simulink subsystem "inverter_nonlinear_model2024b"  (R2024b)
settings: Solver=VariableStepAuto  StartTime=0.0  StopTime=10.0  RelTol=1e-3
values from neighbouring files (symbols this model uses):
  Cdc = diag(Cdc1.*ones(nv,1))    [nine_bus_parameters.m]
  Cf = diag(Cf1.*ones(nv,1))    [nine_bus_parameters.m]
  F = diag(F1.*ones(nv,1))    [nine_bus_parameters.m]
  Kic = diag(Kic1.*ones(nv,1))    [nine_bus_parameters.m]
  Kiv = diag(Kiv1.*ones(nv,1))    [nine_bus_parameters.m]
  Kpc = diag(Kpc1.*ones(nv,1))    [nine_bus_parameters.m]
  Kpv = diag(Kpv1.*ones(nv,1))    [nine_bus_parameters.m]
  Lc = diag(Lc1.*ones(nv,1))    [nine_bus_parameters.m]
  Ldc = diag(Ldc1.*ones(nv,1))    [nine_bus_parameters.m]
  Lf = diag(Lf1.*ones(nv,1))    [nine_bus_parameters.m]
  mp = diag(mp1.*ones(nv,1))    [nine_bus_parameters.m]
  nq = diag(nq1.*ones(nv,1))    [nine_bus_parameters.m]
  rc = diag(rc1.*ones(nv,1))    [nine_bus_parameters.m]
  rdc = diag(rdc1.*ones(nv,1))    [nine_bus_parameters.m]
  rf = diag(rf1.*ones(nv,1))    [nine_bus_parameters.m]
  Vdc = ones(num_inv,1).*Vdc(1)    [nine_bus_initial_conditions.m]    (also in nine_bus_parameters.m = Vdc1.*ones(nv,1))
  Vn = 380    [simulink_parameters_one_bus.m]    (also in nine_bus_parameters.m = 310.*ones(num_inv,1))
  Vtri = Vdc1./3    [simulink_parameters_one_bus.m]    (also in nine_bus_parameters.m = Vdc./2)
  wc = diag(wc1.*ones(nv,1))    [nine_bus_parameters.m]
  wn = ones(num_inv,1).*w01    [nine_bus_parameters.m]    (also in computeModeFrequencyDampingTable.m = abs(lambda))
  x0 = x01    [mlinearize_noninv.m]    (also in onebus_nonlinsub.m; DemoMTI_Boolean_Index_MTI.m = [0.5 0.0000]; DemoMTI_EKF.m = [1;-1;0.5]; DemoMTI_hybridSystemsTankExamples.m = 30)
libraries: slpidlib x4

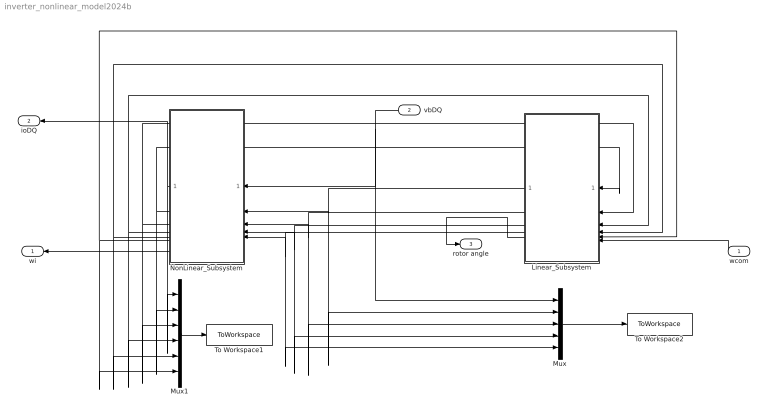
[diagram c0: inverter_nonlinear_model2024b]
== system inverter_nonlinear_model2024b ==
  wcom : Inport
  vbDQ : Inport  Port=2  OutDataTypeStr=double  PortDimensions=2
  Linear_Subsystem : Subsystem
  Mux : Mux  Inputs=5
  Mux1 : Mux  Inputs=6
  NonLinear_Subsystem : Subsystem
  To Workspace1 : ToWorkspace  VariableName=output_data  SaveFormat=Timeseries  SampleTime=-1
  To Workspace2 : ToWorkspace  VariableName=input_data  SaveFormat=Timeseries  SampleTime=-1
  wi : Outport
  ioDQ : Outport  Port=2
  rotor angle : Outport  Port=3
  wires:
  wcom/1 -> Linear_Subsystem/6(wcom)
  Linear_Subsystem/3(wi) -> Mux/4, NonLinear_Subsystem/4(wi_in)
  vbDQ/1 -> Mux/1, NonLinear_Subsystem/1(vbDQ)
  Linear_Subsystem/1(P) -> Mux/2, NonLinear_Subsystem/2(P)
  Linear_Subsystem/2(vref) -> Mux/3, NonLinear_Subsystem/3(vref)
  Linear_Subsystem/4(delta) -> Mux/5, NonLinear_Subsystem/5(delta)
  NonLinear_Subsystem/1(ioDQ) -> ioDQ/1, Mux1/1
  NonLinear_Subsystem/2(il) -> Linear_Subsystem/1(il), Mux1/2
  NonLinear_Subsystem/3(io) -> Linear_Subsystem/2(io), Mux1/3
  NonLinear_Subsystem/4(vo) -> Linear_Subsystem/3(vo), Mux1/4
  NonLinear_Subsystem/5(p) -> Mux1/5, Linear_Subsystem/4(p)
  NonLinear_Subsystem/6(q) -> Linear_Subsystem/5(q), Mux1/6
  Mux/1 -> To Workspace2/1
  NonLinear_Subsystem/7(wi_out) -> wi/1
  Linear_Subsystem/5(rotor angle) -> rotor angle/1
  Mux1/1 -> To Workspace1/1

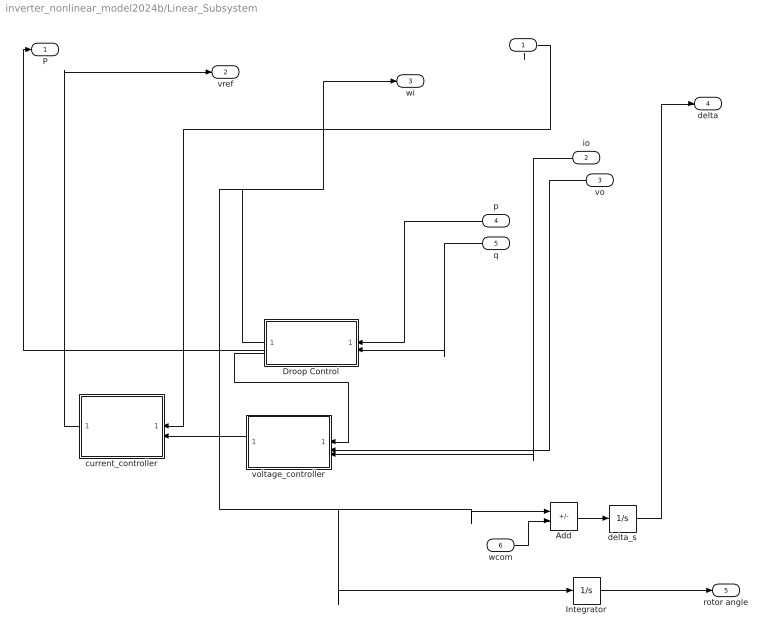
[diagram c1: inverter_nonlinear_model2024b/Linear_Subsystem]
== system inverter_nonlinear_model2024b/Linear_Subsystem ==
  il : Inport
  io : Inport  Port=2
  vo : Inport  Port=3
  p : Inport  Port=4
  q : Inport  Port=5
  wcom : Inport  Port=6
  Add : Sum  Inputs=+-
  Droop Control : Subsystem
  Integrator : Integrator  InitialCondition=2*pi*60  ZeroCross=off
  current_controller : Subsystem
  delta_s : Integrator  InitialCondition=x0(3)
  voltage_controller : Subsystem
  P : Outport
  vref : Outport  Port=2
  wi : Outport  Port=3
  delta : Outport  Port=4
  rotor angle : Outport  Port=5  VectorParamsAs1DForOutWhenUnconnected=off
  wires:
  Droop Control/1(wi) -> wi/1, Add/1, Integrator/1
  Integrator/1 -> rotor angle/1
  Droop Control/2(P) -> P/1
  Droop Control/3(voref) -> voltage_controller/1(voref)
  Add/1 -> delta_s/1
  vo/1 -> voltage_controller/2(vo)
  voltage_controller/1(iref) -> current_controller/2(ilref)
  wcom/1 -> Add/2
  p/1 -> Droop Control/1(p)
  q/1 -> Droop Control/2(q)
  il/1 -> current_controller/1(il)
  current_controller/1(vref) -> vref/1
  delta_s/1 -> delta/1
  io/1 -> voltage_controller/3(io)

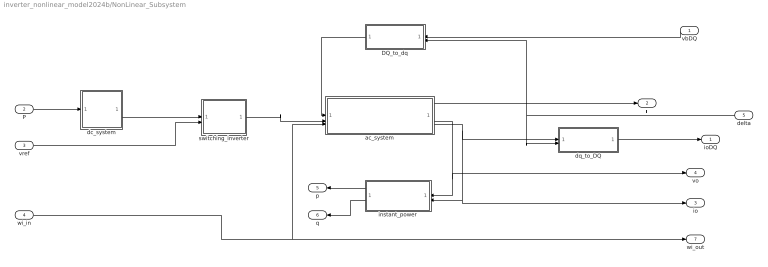
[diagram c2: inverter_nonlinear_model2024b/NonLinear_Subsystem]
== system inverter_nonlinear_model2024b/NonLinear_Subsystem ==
  vbDQ : Inport
  P : Inport  Port=2
  vref : Inport  Port=3
  wi_in : Inport  Port=4
  delta : Inport  Port=5
  DQ_to_dq : MATLAB Function  TreatAsAtomicUnit=on
  ac_system : Subsystem
  dc_system : Subsystem
  dq_to_DQ : MATLAB Function  TreatAsAtomicUnit=on
  instant_power : Subsystem
  switching_inverter : Subsystem
  ioDQ : Outport
  il : Outport  Port=2
  io : Outport  Port=3
  vo : Outport  Port=4
  p : Outport  Port=5
  q : Outport  Port=6
  wi_out : Outport  Port=7
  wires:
  ac_system/3(io) -> io/1, instant_power/2(io), dq_to_DQ/1(iodq)
  dc_system/1(vdc) -> switching_inverter/1(vdc)
  delta/1 -> dq_to_DQ/2(delta), DQ_to_dq/2(delta)
  DQ_to_dq/1(vbdq) -> ac_system/1(vb)
  switching_inverter/1(vl) -> ac_system/2(vl)
  instant_power/2(q) -> q/1
  vbDQ/1 -> DQ_to_dq/1(vbDQ)
  instant_power/1(p) -> p/1
  ac_system/2(vo) -> instant_power/1(vo), vo/1
  ac_system/1(il) -> il/1
  dq_to_DQ/1(ioDQ) -> ioDQ/1
  wi_in/1 -> ac_system/3(wi), wi_out/1
  P/1 -> dc_system/1(P)
  vref/1 -> switching_inverter/2(vref)

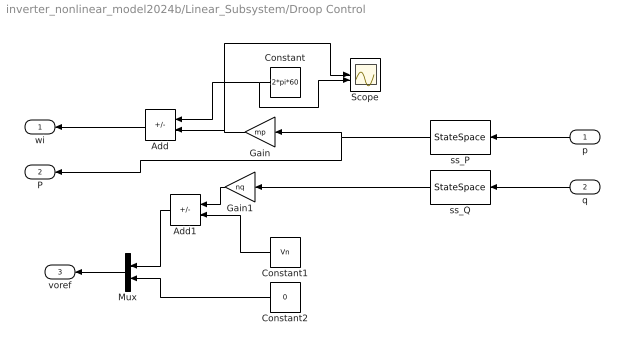
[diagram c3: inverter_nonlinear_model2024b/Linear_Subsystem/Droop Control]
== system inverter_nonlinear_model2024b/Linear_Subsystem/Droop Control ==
  p : Inport
  q : Inport  Port=2
  Add : Sum  Inputs=+-
  Add1 : Sum  Inputs=-+
  Constant : Constant  Value=2*pi*60
  Constant1 : Constant  Value=Vn
  Constant2 : Constant  Value=0
  Gain : Gain  Gain=mp
  Gain1 : Gain  Gain=nq
  Mux : Mux  Inputs=2
  Scope : Scope  NumInputPorts=2
  ss_P : StateSpace  A=-wc  B=wc  D=0  InitialCondition=x0(4)
  ss_Q : StateSpace  A=-wc  B=wc  D=0  InitialCondition=x0(5)
  wi : Outport
  P : Outport  Port=2
  voref : Outport  Port=3
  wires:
  ss_P/1 -> P/1, Gain/1
  Constant1/1 -> Add1/2
  ss_Q/1 -> Gain1/1
  Gain/1 -> Scope/1, Add/2
  Mux/1 -> voref/1
  Add1/1 -> Mux/1
  Constant/1 -> Scope/2, Add/1
  Constant2/1 -> Mux/2
  Gain1/1 -> Add1/1
  q/1 -> ss_Q/1
  p/1 -> ss_P/1
  Add/1 -> wi/1

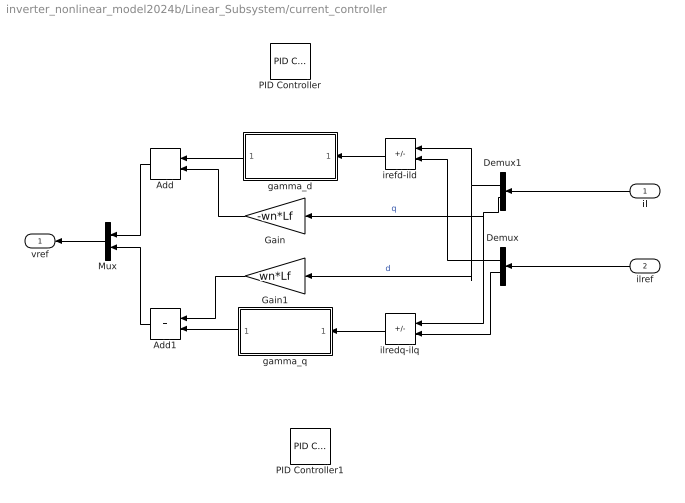
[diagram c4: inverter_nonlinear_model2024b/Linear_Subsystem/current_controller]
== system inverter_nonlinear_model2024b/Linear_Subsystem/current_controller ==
  il : Inport
  ilref : Inport  Port=2
  Add : Sum
  Add1 : Sum
  Demux : Demux  Outputs=2
  Demux1 : Demux  Outputs=2
  Gain : Gain  Gain=-wn*Lf
  Gain1 : Gain  Gain=wn*Lf
  Mux : Mux  Inputs=2
  PID Controller : slpidlib/PID Controller  Commented=on  Controller=PI  Form=Parallel  TimeDomain=Continuous-time  UseExternalTs=off  SampleTime=-1  IntegratorMethod=Forward Euler  FilterMethod=Forward Euler  ControllerParametersSource=internal  P=Kpc  I=Kic  UseKiTs=off  D=0  UseExternalDerivativeSource=off  N=100  UseFilter=on  TunerSelectOption=Transfer Function Based (PID Tuner App)  InitialConditionSource=internal  InitialConditionForIntegrator=x0(8)  InitialConditionForFilter=0  DifferentiatorICPrevScaledInput=0  ExternalReset=none  TrackingMode=off  Kt=1  LimitOutput=off  SatLimitsSource=internal  UpperSaturationLimit=inf  LowerSaturationLimit=-inf  LinearizeAsGain=on  AntiWindupMode=none  Kb=1  LimitIntegrator=off  UpperIntegratorSaturationLimit=inf  LowerIntegratorSaturationLimit=-inf  POutMin=[]  POutMax=[]  IOutMin=[]  IOutMax=[]  DOutMin=[]  DOutMax=[]  NOutMin=[]  NOutMax=[]  SumOutMin=[]  SumOutMax=[]  SaturationOutMin=[]  SaturationOutMax=[]  PParamMin=[]  PParamMax=[]  IParamMin=[]  IParamMax=[]  DParamMin=[]  DParamMax=[]  NParamMin=[]  NParamMax=[]  KbParamMin=[]  KbParamMax=[]  KtParamMin=[]  KtParamMax=[]  KbOutMin=[]  KbOutMax=[]  KtOutMin=[]  KtOutMax=[]  IntegratorOutMin=[]  IntegratorOutMax=[]  FilterOutMin=[]  FilterOutMax=[]  SumI1OutMin=[]  SumI1OutMax=[]  SumI2OutMin=[]  SumI2OutMax=[]  SumI3OutMin=[]  SumI3OutMax=[]  SumI4OutMin=[]  SumI4OutMax=[]  SumDOutMin=[]  SumDOutMax=[]  DifferentiatorOutMin=[]  DifferentiatorOutMax=[]  FilterDiffOutCoefMin=[]  FilterDiffOutCoefMax=[]  ReciprocalOutMin=[]  ReciprocalOutMax=[]  SumDenOutMin=[]  SumDenOutMax=[]  SumNumOutMin=[]  SumNumOutMax=[]  DivideOutMin=[]  DivideOutMax=[]  UdiffTsProdOutMin=[]  UdiffTsProdOutMax=[]  NTsProdOutMin=[]  NTsProdOutMax=[]  UintegralTsProdOutMin=[]  UintegralTsProdOutMax=[]  UngainTsProdOutMin=[]  UngainTsProdOutMax=[]  ClampingZeroOutDataTypeStr=Inherit: Inherit via back propagation  ClampingZeroOutMin=[]  ClampingZeroOutMax=[]  FilterDenConstantOutDataTypeStr=Inherit: Inherit via back propagation  FilterDenConstantOutMin=[]  FilterDenConstantOutMax=[]  PCopyOutDataTypeStr=Inherit: Inherit via back propagation  PCopyOutMin=[]  PCopyOutMax=[]  NCopyOutDataTypeStr=Inherit: Inherit via back propagation  NCopyOutMin=[]  NCopyOutMax=[]  IntegratorContinuousStateAttributes=''  IntegratorStateMustResolveToSignalObject=off  IntegratorRTWStateStorageClass=Auto  FilterContinuousStateAttributes=''  FilterStateMustResolveToSignalObject=off  FilterRTWStateStorageClass=Auto  ParallelPVariant=InternalParameters  IdealPVariant=Disabled  IVariant=InternalParameters  DVariant=Disabled  IntegratorVariant=Continuous  SatVariant=Disabled  AWVariant=Passthrough  PCopyVariant=Disabled  TRVariant=Disabled  FdbkBlocksVariant=Forward  IdealPFdbkVariant=Disabled  SatFdbkVariant=Disabled  DerivativeFilterVariant=Disabled  NVariant=Disabled  NCopyVariant=Disabled_SignalSpec  FilterICVariant=Disabled  IntegratorICVariant=InternalICs  ExternalResetVariant=Disabled  TRSumVariant=Passthrough  SumFdbkVariant=Disabled  SumVariant=Sum_PI  TsampFilterVariant=InternalTs  TsampNgainVariant=Passthrough  TsampIntegralVariant=Disabled_SignalSpec  ExternalSaturationOutDataTypeStr=Inherit: Same as second input  DerivativeSourceVariant=Disabled  PreIntVariant=InternalPreInt
  PID Controller1 : slpidlib/PID Controller  Commented=on  Controller=PI  Form=Parallel  TimeDomain=Continuous-time  UseExternalTs=off  SampleTime=-1  IntegratorMethod=Forward Euler  FilterMethod=Forward Euler  ControllerParametersSource=internal  P=Kpc  I=Kic  UseKiTs=off  D=0  UseExternalDerivativeSource=off  N=100  UseFilter=on  TunerSelectOption=Transfer Function Based (PID Tuner App)  InitialConditionSource=internal  InitialConditionForIntegrator=x0(9)  InitialConditionForFilter=0  DifferentiatorICPrevScaledInput=0  ExternalReset=none  TrackingMode=off  Kt=1  LimitOutput=off  SatLimitsSource=internal  UpperSaturationLimit=inf  LowerSaturationLimit=-inf  LinearizeAsGain=on  AntiWindupMode=none  Kb=1  LimitIntegrator=off  UpperIntegratorSaturationLimit=inf  LowerIntegratorSaturationLimit=-inf  POutMin=[]  POutMax=[]  IOutMin=[]  IOutMax=[]  DOutMin=[]  DOutMax=[]  NOutMin=[]  NOutMax=[]  SumOutMin=[]  SumOutMax=[]  SaturationOutMin=[]  SaturationOutMax=[]  PParamMin=[]  PParamMax=[]  IParamMin=[]  IParamMax=[]  DParamMin=[]  DParamMax=[]  NParamMin=[]  NParamMax=[]  KbParamMin=[]  KbParamMax=[]  KtParamMin=[]  KtParamMax=[]  KbOutMin=[]  KbOutMax=[]  KtOutMin=[]  KtOutMax=[]  IntegratorOutMin=[]  IntegratorOutMax=[]  FilterOutMin=[]  FilterOutMax=[]  SumI1OutMin=[]  SumI1OutMax=[]  SumI2OutMin=[]  SumI2OutMax=[]  SumI3OutMin=[]  SumI3OutMax=[]  SumI4OutMin=[]  SumI4OutMax=[]  SumDOutMin=[]  SumDOutMax=[]  DifferentiatorOutMin=[]  DifferentiatorOutMax=[]  FilterDiffOutCoefMin=[]  FilterDiffOutCoefMax=[]  ReciprocalOutMin=[]  ReciprocalOutMax=[]  SumDenOutMin=[]  SumDenOutMax=[]  SumNumOutMin=[]  SumNumOutMax=[]  DivideOutMin=[]  DivideOutMax=[]  UdiffTsProdOutMin=[]  UdiffTsProdOutMax=[]  NTsProdOutMin=[]  NTsProdOutMax=[]  UintegralTsProdOutMin=[]  UintegralTsProdOutMax=[]  UngainTsProdOutMin=[]  UngainTsProdOutMax=[]  ClampingZeroOutDataTypeStr=Inherit: Inherit via back propagation  ClampingZeroOutMin=[]  ClampingZeroOutMax=[]  FilterDenConstantOutDataTypeStr=Inherit: Inherit via back propagation  FilterDenConstantOutMin=[]  FilterDenConstantOutMax=[]  PCopyOutDataTypeStr=Inherit: Inherit via back propagation  PCopyOutMin=[]  PCopyOutMax=[]  NCopyOutDataTypeStr=Inherit: Inherit via back propagation  NCopyOutMin=[]  NCopyOutMax=[]  IntegratorContinuousStateAttributes=''  IntegratorStateMustResolveToSignalObject=off  IntegratorRTWStateStorageClass=Auto  FilterContinuousStateAttributes=''  FilterStateMustResolveToSignalObject=off  FilterRTWStateStorageClass=Auto  ParallelPVariant=InternalParameters  IdealPVariant=Disabled  IVariant=InternalParameters  DVariant=Disabled  IntegratorVariant=Continuous  SatVariant=Disabled  AWVariant=Passthrough  PCopyVariant=Disabled  TRVariant=Disabled  FdbkBlocksVariant=Forward  IdealPFdbkVariant=Disabled  SatFdbkVariant=Disabled  DerivativeFilterVariant=Disabled  NVariant=Disabled  NCopyVariant=Disabled_SignalSpec  FilterICVariant=Disabled  IntegratorICVariant=InternalICs  ExternalResetVariant=Disabled  TRSumVariant=Passthrough  SumFdbkVariant=Disabled  SumVariant=Sum_PI  TsampFilterVariant=InternalTs  TsampNgainVariant=Passthrough  TsampIntegralVariant=Disabled_SignalSpec  ExternalSaturationOutDataTypeStr=Inherit: Same as second input  DerivativeSourceVariant=Disabled  PreIntVariant=InternalPreInt
  gamma_d : Subsystem
  gamma_q : Subsystem
  ilredq-ilq : Sum  Inputs=-+
  irefd-ild : Sum  Inputs=-+
  vref : Outport
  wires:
  Add1/1 -> Mux/2
  Demux1/2 -> Gain/1, ilredq-ilq/1  "q"
  Demux/1 -> irefd-ild/2
  Add/1 -> Mux/1
  il/1 -> Demux1/1
  Mux/1 -> vref/1
  Gain1/1 -> Add1/1
  Gain/1 -> Add/2
  Demux1/1 -> Gain1/1, irefd-ild/1  "d"
  Demux/2 -> ilredq-ilq/2
  ilref/1 -> Demux/1
  irefd-ild/1 -> gamma_d/1(In1)
  gamma_d/1(Out1) -> Add/1
  gamma_q/1(Out1) -> Add1/2
  ilredq-ilq/1 -> gamma_q/1(In1)

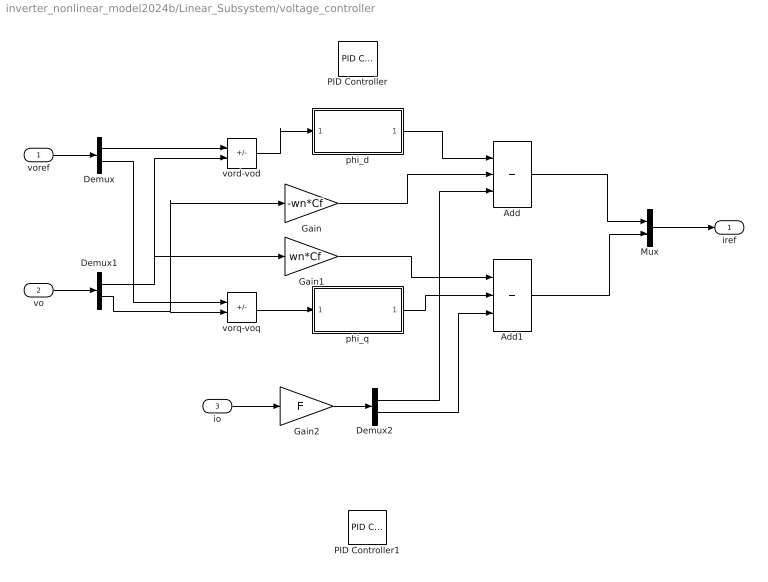
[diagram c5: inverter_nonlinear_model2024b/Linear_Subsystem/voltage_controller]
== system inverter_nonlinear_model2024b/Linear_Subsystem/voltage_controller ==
  voref : Inport
  vo : Inport  Port=2
  io : Inport  Port=3
  Add : Sum  Inputs=+++
  Add1 : Sum  Inputs=+++
  Demux : Demux  Outputs=2
  Demux1 : Demux  Outputs=2
  Demux2 : Demux  Outputs=2
  Gain : Gain  Gain=-wn*Cf
  Gain1 : Gain  Gain=wn*Cf
  Gain2 : Gain  Gain=F
  Mux : Mux  Inputs=2
  PID Controller : slpidlib/PID Controller  Commented=on  Controller=PI  Form=Parallel  TimeDomain=Continuous-time  UseExternalTs=off  SampleTime=-1  IntegratorMethod=Forward Euler  FilterMethod=Forward Euler  ControllerParametersSource=internal  P=Kpv  I=Kiv  UseKiTs=off  D=0  UseExternalDerivativeSource=off  N=100  UseFilter=on  TunerSelectOption=Transfer Function Based (PID Tuner App)  InitialConditionSource=internal  InitialConditionForIntegrator=x0(6)  InitialConditionForFilter=0  DifferentiatorICPrevScaledInput=0  ExternalReset=none  TrackingMode=off  Kt=1  LimitOutput=off  SatLimitsSource=internal  UpperSaturationLimit=inf  LowerSaturationLimit=-inf  LinearizeAsGain=on  AntiWindupMode=none  Kb=1  LimitIntegrator=off  UpperIntegratorSaturationLimit=inf  LowerIntegratorSaturationLimit=-inf  POutMin=[]  POutMax=[]  IOutMin=[]  IOutMax=[]  DOutMin=[]  DOutMax=[]  NOutMin=[]  NOutMax=[]  SumOutMin=[]  SumOutMax=[]  SaturationOutMin=[]  SaturationOutMax=[]  PParamMin=[]  PParamMax=[]  IParamMin=[]  IParamMax=[]  DParamMin=[]  DParamMax=[]  NParamMin=[]  NParamMax=[]  KbParamMin=[]  KbParamMax=[]  KtParamMin=[]  KtParamMax=[]  KbOutMin=[]  KbOutMax=[]  KtOutMin=[]  KtOutMax=[]  IntegratorOutMin=[]  IntegratorOutMax=[]  FilterOutMin=[]  FilterOutMax=[]  SumI1OutMin=[]  SumI1OutMax=[]  SumI2OutMin=[]  SumI2OutMax=[]  SumI3OutMin=[]  SumI3OutMax=[]  SumI4OutMin=[]  SumI4OutMax=[]  SumDOutMin=[]  SumDOutMax=[]  DifferentiatorOutMin=[]  DifferentiatorOutMax=[]  FilterDiffOutCoefMin=[]  FilterDiffOutCoefMax=[]  ReciprocalOutMin=[]  ReciprocalOutMax=[]  SumDenOutMin=[]  SumDenOutMax=[]  SumNumOutMin=[]  SumNumOutMax=[]  DivideOutMin=[]  DivideOutMax=[]  UdiffTsProdOutMin=[]  UdiffTsProdOutMax=[]  NTsProdOutMin=[]  NTsProdOutMax=[]  UintegralTsProdOutMin=[]  UintegralTsProdOutMax=[]  UngainTsProdOutMin=[]  UngainTsProdOutMax=[]  ClampingZeroOutDataTypeStr=Inherit: Inherit via back propagation  ClampingZeroOutMin=[]  ClampingZeroOutMax=[]  FilterDenConstantOutDataTypeStr=Inherit: Inherit via back propagation  FilterDenConstantOutMin=[]  FilterDenConstantOutMax=[]  PCopyOutDataTypeStr=Inherit: Inherit via back propagation  PCopyOutMin=[]  PCopyOutMax=[]  NCopyOutDataTypeStr=Inherit: Inherit via back propagation  NCopyOutMin=[]  NCopyOutMax=[]  IntegratorContinuousStateAttributes=''  IntegratorStateMustResolveToSignalObject=off  IntegratorRTWStateStorageClass=Auto  FilterContinuousStateAttributes=''  FilterStateMustResolveToSignalObject=off  FilterRTWStateStorageClass=Auto  ParallelPVariant=InternalParameters  IdealPVariant=Disabled  IVariant=InternalParameters  DVariant=Disabled  IntegratorVariant=Continuous  SatVariant=Disabled  AWVariant=Passthrough  PCopyVariant=Disabled  TRVariant=Disabled  FdbkBlocksVariant=Forward  IdealPFdbkVariant=Disabled  SatFdbkVariant=Disabled  DerivativeFilterVariant=Disabled  NVariant=Disabled  NCopyVariant=Disabled_SignalSpec  FilterICVariant=Disabled  IntegratorICVariant=InternalICs  ExternalResetVariant=Disabled  TRSumVariant=Passthrough  SumFdbkVariant=Disabled  SumVariant=Sum_PI  TsampFilterVariant=InternalTs  TsampNgainVariant=Passthrough  TsampIntegralVariant=Disabled_SignalSpec  ExternalSaturationOutDataTypeStr=Inherit: Same as second input  DerivativeSourceVariant=Disabled  PreIntVariant=InternalPreInt
  PID Controller1 : slpidlib/PID Controller  Commented=on  Controller=PI  Form=Parallel  TimeDomain=Continuous-time  UseExternalTs=off  SampleTime=-1  IntegratorMethod=Forward Euler  FilterMethod=Forward Euler  ControllerParametersSource=internal  P=Kpv  I=Kiv  UseKiTs=off  D=0  UseExternalDerivativeSource=off  N=100  UseFilter=on  TunerSelectOption=Frequency Response Based  InitialConditionSource=internal  InitialConditionForIntegrator=x0(7)  InitialConditionForFilter=0  DifferentiatorICPrevScaledInput=0  ExternalReset=none  TrackingMode=off  Kt=1  LimitOutput=off  SatLimitsSource=internal  UpperSaturationLimit=inf  LowerSaturationLimit=-inf  LinearizeAsGain=on  AntiWindupMode=none  Kb=1  LimitIntegrator=off  UpperIntegratorSaturationLimit=inf  LowerIntegratorSaturationLimit=-inf  POutMin=[]  POutMax=[]  IOutMin=[]  IOutMax=[]  DOutMin=[]  DOutMax=[]  NOutMin=[]  NOutMax=[]  SumOutMin=[]  SumOutMax=[]  SaturationOutMin=[]  SaturationOutMax=[]  PParamMin=[]  PParamMax=[]  IParamMin=[]  IParamMax=[]  DParamMin=[]  DParamMax=[]  NParamMin=[]  NParamMax=[]  KbParamMin=[]  KbParamMax=[]  KtParamMin=[]  KtParamMax=[]  KbOutMin=[]  KbOutMax=[]  KtOutMin=[]  KtOutMax=[]  IntegratorOutMin=[]  IntegratorOutMax=[]  FilterOutMin=[]  FilterOutMax=[]  SumI1OutMin=[]  SumI1OutMax=[]  SumI2OutMin=[]  SumI2OutMax=[]  SumI3OutMin=[]  SumI3OutMax=[]  SumI4OutMin=[]  SumI4OutMax=[]  SumDOutMin=[]  SumDOutMax=[]  DifferentiatorOutMin=[]  DifferentiatorOutMax=[]  FilterDiffOutCoefMin=[]  FilterDiffOutCoefMax=[]  ReciprocalOutMin=[]  ReciprocalOutMax=[]  SumDenOutMin=[]  SumDenOutMax=[]  SumNumOutMin=[]  SumNumOutMax=[]  DivideOutMin=[]  DivideOutMax=[]  UdiffTsProdOutMin=[]  UdiffTsProdOutMax=[]  NTsProdOutMin=[]  NTsProdOutMax=[]  UintegralTsProdOutMin=[]  UintegralTsProdOutMax=[]  UngainTsProdOutMin=[]  UngainTsProdOutMax=[]  ClampingZeroOutDataTypeStr=Inherit: Inherit via back propagation  ClampingZeroOutMin=[]  ClampingZeroOutMax=[]  FilterDenConstantOutDataTypeStr=Inherit: Inherit via back propagation  FilterDenConstantOutMin=[]  FilterDenConstantOutMax=[]  PCopyOutDataTypeStr=Inherit: Inherit via back propagation  PCopyOutMin=[]  PCopyOutMax=[]  NCopyOutDataTypeStr=Inherit: Inherit via back propagation  NCopyOutMin=[]  NCopyOutMax=[]  IntegratorContinuousStateAttributes=''  IntegratorStateMustResolveToSignalObject=off  IntegratorRTWStateStorageClass=Auto  FilterContinuousStateAttributes=''  FilterStateMustResolveToSignalObject=off  FilterRTWStateStorageClass=Auto  ParallelPVariant=InternalParameters  IdealPVariant=Disabled  IVariant=InternalParameters  DVariant=Disabled  IntegratorVariant=Continuous  SatVariant=Disabled  AWVariant=Passthrough  PCopyVariant=Disabled  TRVariant=Disabled  FdbkBlocksVariant=Forward  IdealPFdbkVariant=Disabled  SatFdbkVariant=Disabled  DerivativeFilterVariant=Disabled  NVariant=Disabled  NCopyVariant=Disabled_SignalSpec  FilterICVariant=Disabled  IntegratorICVariant=InternalICs  ExternalResetVariant=Disabled  TRSumVariant=Passthrough  SumFdbkVariant=Disabled  SumVariant=Sum_PI  TsampFilterVariant=InternalTs  TsampNgainVariant=Passthrough  TsampIntegralVariant=Disabled_SignalSpec  ExternalSaturationOutDataTypeStr=Inherit: Same as second input  DerivativeSourceVariant=Disabled  PreIntVariant=InternalPreInt
  phi_d : Subsystem
  phi_q : Subsystem
  vord-vod : Sum  Inputs=+-
  vorq-voq : Sum  Inputs=+-
  iref : Outport
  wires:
  Gain2/1 -> Demux2/1
  Add/1 -> Mux/1
  Demux2/2 -> Add1/3
  Gain/1 -> Add/2
  Gain1/1 -> Add1/1
  Mux/1 -> iref/1
  Demux1/1 -> Gain1/1, vord-vod/2
  Demux1/2 -> Gain/1, vorq-voq/2
  Demux2/1 -> Add/3
  voref/1 -> Demux/1
  vo/1 -> Demux1/1
  io/1 -> Gain2/1
  Demux/2 -> vorq-voq/1
  Demux/1 -> vord-vod/1
  Add1/1 -> Mux/2
  vord-vod/1 -> phi_d/1(In1)
  phi_d/1(Out1) -> Add/1
  vorq-voq/1 -> phi_q/1(In1)
  phi_q/1(Out1) -> Add1/2

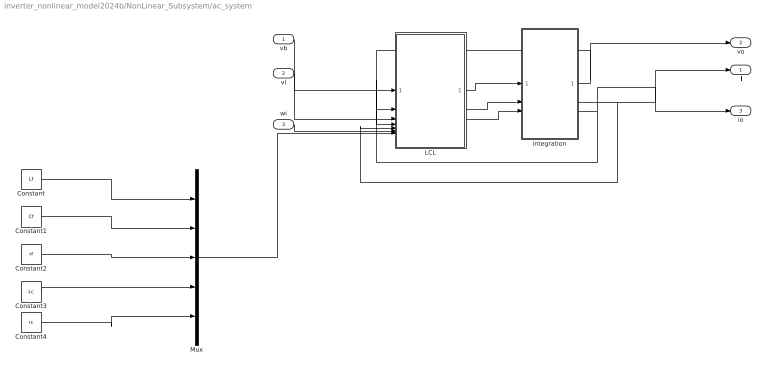
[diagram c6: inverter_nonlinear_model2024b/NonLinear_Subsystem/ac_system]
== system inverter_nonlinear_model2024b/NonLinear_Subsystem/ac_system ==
  vb : Inport
  vl : Inport  Port=2
  wi : Inport  Port=3
  Constant : Constant  Value=Lf
  Constant1 : Constant  Value=Cf
  Constant2 : Constant  Value=rf
  Constant3 : Constant  Value=Lc
  Constant4 : Constant  Value=rc
  LCL : MATLAB Function  TreatAsAtomicUnit=on
  Mux : Mux  Inputs=5
  integration : Subsystem
  il : Outport  PortDimensions=[2 1]
  vo : Outport  Port=2  PortDimensions=[2 1]
  io : Outport  Port=3  PortDimensions=[2 1]
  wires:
  vl/1 -> LCL/3(vl)
  vb/1 -> LCL/1(vb)
  wi/1 -> LCL/6(wi)
  LCL/1(dil) -> integration/1(dil)
  LCL/2(dio) -> integration/2(dio)
  LCL/3(dvo) -> integration/3(dvo)
  integration/2(il) -> LCL/5(il), il/1
  integration/3(io) -> io/1, LCL/4(io)
  integration/1(vo) -> vo/1, LCL/2(vo)
  Constant/1 -> Mux/1
  Constant1/1 -> Mux/2
  Constant2/1 -> Mux/3
  Constant3/1 -> Mux/4
  Constant4/1 -> Mux/5
  Mux/1 -> LCL/7(params)

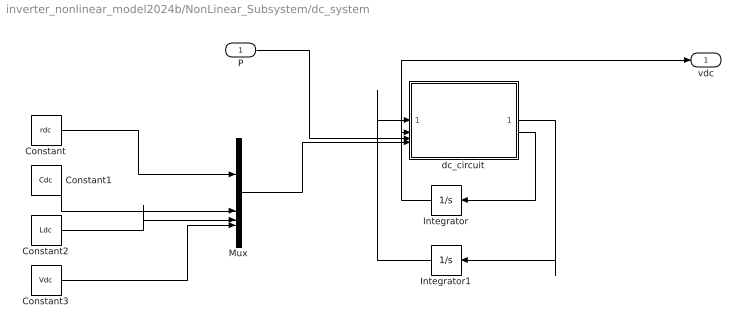
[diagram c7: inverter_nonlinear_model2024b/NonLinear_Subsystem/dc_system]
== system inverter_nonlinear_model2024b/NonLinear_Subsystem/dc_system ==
  P : Inport
  Constant : Constant  Value=rdc
  Constant1 : Constant  Value=Cdc
  Constant2 : Constant  Value=Ldc
  Constant3 : Constant  Value=Vdc
  Integrator : Integrator  InitialCondition=x0(2)
  Integrator1 : Integrator  InitialCondition=x0(1)
  Mux : Mux
  dc_circuit : MATLAB Function  TreatAsAtomicUnit=on
  vdc : Outport  PortDimensions=1
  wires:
  dc_circuit/1(didc) -> Integrator1/1
  Integrator1/1 -> dc_circuit/1(idc)
  P/1 -> dc_circuit/3(P)
  dc_circuit/2(dvdc) -> Integrator/1
  Integrator/1 -> vdc/1, dc_circuit/2(vdc)
  Constant/1 -> Mux/1
  Mux/1 -> dc_circuit/4(params)
  Constant1/1 -> Mux/2
  Constant2/1 -> Mux/3
  Constant3/1 -> Mux/4

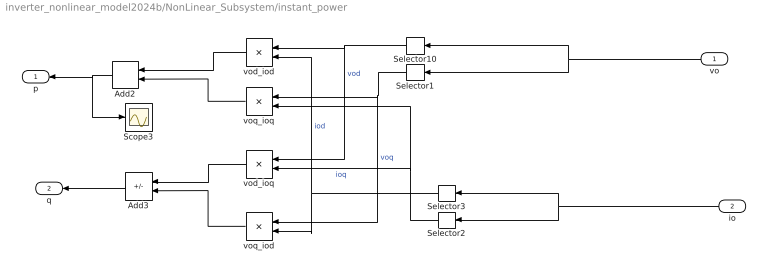
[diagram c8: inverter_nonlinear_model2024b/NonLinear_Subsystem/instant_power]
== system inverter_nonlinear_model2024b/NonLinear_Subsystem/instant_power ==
  vo : Inport
  io : Inport  Port=2
  Add2 : Sum
  Add3 : Sum  Inputs=+-
  Scope3 : Scope
  Selector1 : Selector  InputPortWidth=2  IndexOptions=Index vector (dialog)  Indices=2  OutputSizes=1
  Selector10 : Selector  InputPortWidth=2  IndexOptions=Index vector (dialog)  Indices=1  OutputSizes=1
  Selector2 : Selector  InputPortWidth=2  IndexOptions=Index vector (dialog)  Indices=2  OutputSizes=1
  Selector3 : Selector  InputPortWidth=2  IndexOptions=Index vector (dialog)  Indices=1  OutputSizes=1
  vod_iod : Product
  vod_ioq : Product
  voq_iod : Product
  voq_ioq : Product
  p : Outport
  q : Outport  Port=2
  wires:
  Selector2/1 -> vod_ioq/2, voq_ioq/2  "ioq"
  vo/1 -> Selector10/1, Selector1/1
  Selector3/1 -> voq_iod/2, vod_iod/2  "iod"
  Selector10/1 -> vod_ioq/1, vod_iod/1  "vod"
  vod_ioq/1 -> Add3/1
  Add2/1 -> p/1, Scope3/1
  voq_iod/1 -> Add3/2
  io/1 -> Selector2/1, Selector3/1
  voq_ioq/1 -> Add2/2
  vod_iod/1 -> Add2/1
  Selector1/1 -> voq_iod/1, voq_ioq/1  "voq"
  Add3/1 -> q/1

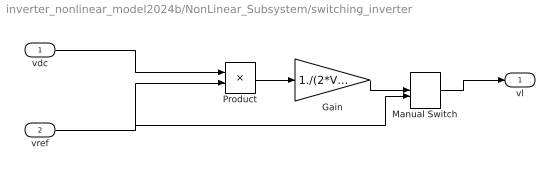
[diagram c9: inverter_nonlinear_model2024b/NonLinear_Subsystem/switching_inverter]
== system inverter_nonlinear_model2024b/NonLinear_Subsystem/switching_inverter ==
  vdc : Inport
  vref : Inport  Port=2
  Gain : Gain  Gain=1./(2*Vtri)
  Manual Switch : ManualSwitch
  Product : Product
  vl : Outport  PortDimensions=[2 1]
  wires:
  Product/1 -> Gain/1
  vdc/1 -> Product/1
  vref/1 -> Manual Switch/2, Product/2
  Gain/1 -> Manual Switch/1
  Manual Switch/1 -> vl/1

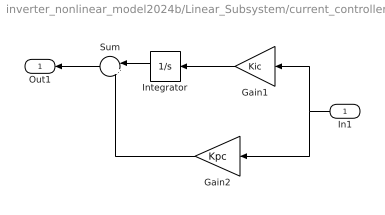
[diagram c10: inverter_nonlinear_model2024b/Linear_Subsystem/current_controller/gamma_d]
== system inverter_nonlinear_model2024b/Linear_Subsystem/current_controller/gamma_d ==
  In1 : Inport
  Gain1 : Gain  Gain=Kic
  Gain2 : Gain  Gain=Kpc
  Integrator : Integrator  InitialCondition=x0(8)
  Sum : Sum  Inputs=|++
  Out1 : Outport
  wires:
  Gain2/1 -> Sum/2
  Integrator/1 -> Sum/1
  In1/1 -> Gain2/1, Gain1/1
  Sum/1 -> Out1/1
  Gain1/1 -> Integrator/1

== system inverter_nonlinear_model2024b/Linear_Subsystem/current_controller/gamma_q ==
  In1 : Inport
  Gain1 : Gain  Gain=Kic
  Gain2 : Gain  Gain=Kpc
  Integrator : Integrator  InitialCondition=x0(9)
  Sum : Sum  Inputs=|++
  Out1 : Outport
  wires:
  Gain2/1 -> Sum/2
  Integrator/1 -> Sum/1
  In1/1 -> Gain2/1, Gain1/1
  Sum/1 -> Out1/1
  Gain1/1 -> Integrator/1

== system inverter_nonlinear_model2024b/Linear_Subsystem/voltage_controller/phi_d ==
  In1 : Inport
  Gain1 : Gain  Gain=Kiv
  Gain2 : Gain  Gain=Kpv
  Integrator : Integrator  InitialCondition=x0(6)
  Sum : Sum  Inputs=|++
  Out1 : Outport
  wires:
  Gain2/1 -> Sum/2
  Integrator/1 -> Sum/1
  In1/1 -> Gain2/1, Gain1/1
  Sum/1 -> Out1/1
  Gain1/1 -> Integrator/1

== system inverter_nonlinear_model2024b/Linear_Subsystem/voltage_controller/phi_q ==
  In1 : Inport
  Gain1 : Gain  Gain=Kiv
  Gain2 : Gain  Gain=Kpv
  Integrator : Integrator  InitialCondition=x0(7)
  Sum : Sum  Inputs=|++
  Out1 : Outport
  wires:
  Gain2/1 -> Sum/2
  Integrator/1 -> Sum/1
  In1/1 -> Gain2/1, Gain1/1
  Sum/1 -> Out1/1
  Gain1/1 -> Integrator/1

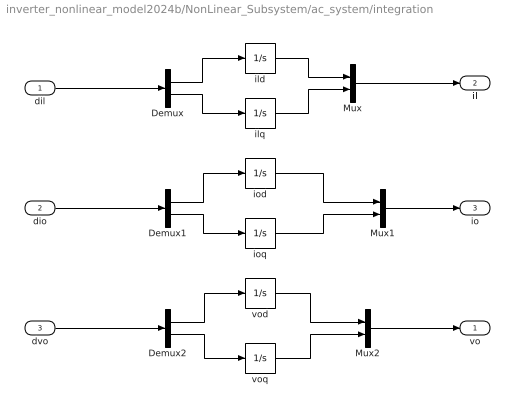
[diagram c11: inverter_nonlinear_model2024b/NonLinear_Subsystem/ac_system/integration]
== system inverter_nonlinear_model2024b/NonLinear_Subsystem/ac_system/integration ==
  dil : Inport
  dio : Inport  Port=2
  dvo : Inport  Port=3
  Demux : Demux  Outputs=2
  Demux1 : Demux  Outputs=2
  Demux2 : Demux  Outputs=2
  Mux : Mux  Inputs=2
  Mux1 : Mux  Inputs=2
  Mux2 : Mux  Inputs=2
  ild : Integrator  InitialCondition=x0(10)
  ilq : Integrator  InitialCondition=x0(11)
  iod : Integrator  InitialCondition=x0(14)
  ioq : Integrator  InitialCondition=x0(15)
  vod : Integrator  InitialCondition=x0(12)
  voq : Integrator  InitialCondition=x0(13)
  vo : Outport
  il : Outport  Port=2
  io : Outport  Port=3
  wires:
  Demux1/1 -> iod/1
  ilq/1 -> Mux/2
  vod/1 -> Mux2/1
  ild/1 -> Mux/1
  voq/1 -> Mux2/2
  ioq/1 -> Mux1/2
  dio/1 -> Demux1/1
  iod/1 -> Mux1/1
  Mux1/1 -> io/1
  Demux2/1 -> vod/1
  Demux2/2 -> voq/1
  Demux1/2 -> ioq/1
  Mux/1 -> il/1
  Mux2/1 -> vo/1
  Demux/1 -> ild/1
  Demux/2 -> ilq/1
  dil/1 -> Demux/1
  dvo/1 -> Demux2/1

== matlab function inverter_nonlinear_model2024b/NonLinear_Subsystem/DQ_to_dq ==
function vbdq  = DQ_to_dq(vbDQ,delta)

vbdq = [cos(delta) sin(delta);-sin(delta) cos(delta)]*vbDQ;

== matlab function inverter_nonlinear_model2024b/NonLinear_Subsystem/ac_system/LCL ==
function [dil,dio,dvo] = ac_circuit(vb,vo,vl,io,il,wi,params)
% 
Lf = params(1);   
Cf = params(2);   
rf = params(3); 
Lc = params(4); 
rc = params(5);

dil = -(rf/Lf).*il + wi.*[0 1;-1 0]*il + (1/Lf).*(vl-vo);
dio = -(rc/Lc).*io + wi.*[0 1;-1 0]*io + (1/Lc).*(vo-vb);
dvo = (1/Cf).*(il-io) + wi.*[0 1;-1 0]*vo;

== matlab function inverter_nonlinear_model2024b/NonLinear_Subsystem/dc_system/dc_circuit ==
function[didc, dvdc] = dc_circuit(idc,vdc,P,params)

% rdc = 28.86;
% Cdc = 5;
% Ldc = 1;
% Vdc = 1000;
rdc = params(1);
Cdc = params(2);
Ldc = params(3);
Vdc = params(4);

dx = [-rdc/Ldc -1/Ldc;1/Cdc 0]*[idc;vdc] + [0;-1/(Cdc*vdc)]*P + [Vdc/Ldc;0];

didc = dx(1);
dvdc = dx(2);

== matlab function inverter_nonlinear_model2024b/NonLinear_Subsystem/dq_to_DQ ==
function ioDQ  = dq_to_DQ(iodq,delta)

ioDQ = [cos(delta) -sin(delta);sin(delta) cos(delta)]*iodq;
